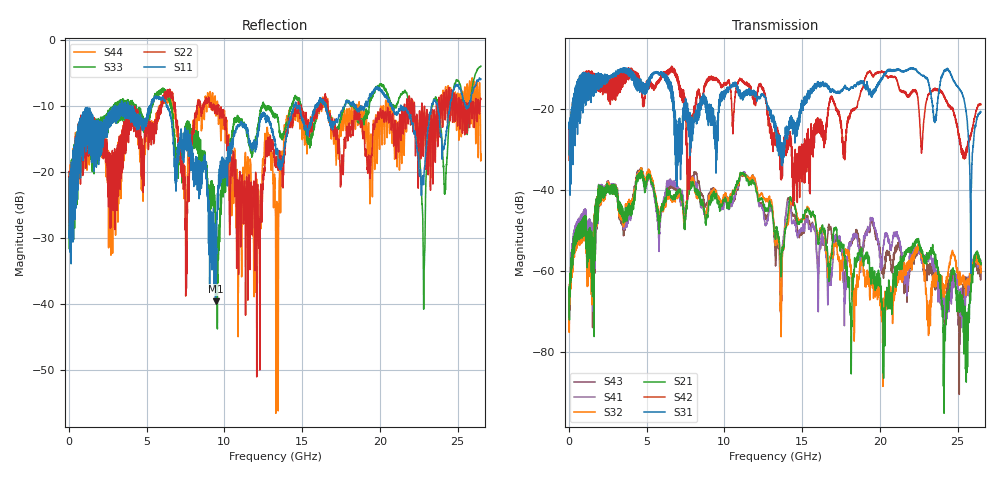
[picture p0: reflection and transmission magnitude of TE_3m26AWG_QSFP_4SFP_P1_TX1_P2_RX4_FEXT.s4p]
!Agilent Technologies,N5222A,MY51421691,A.10.00.00
!Agilent N5222A: A.10.00.00
!Date: Friday, January 30, 2015 12:38:07
!Correction: S11(Full 4 Port(1,2,3,4))
!S12(Full 4 Port(1,2,3,4))
!S13(Full 4 Port(1,2,3,4))
!S14(Full 4 Port(1,2,3,4))
!S21(Full 4 Port(1,2,3,4))
!S22(Full 4 Port(1,2,3,4))
!S23(Full 4 Port(1,2,3,4))
!S24(Full 4 Port(1,2,3,4))
!S31(Full 4 Port(1,2,3,4))
!S32(Full 4 Port(1,2,3,4))
!S33(Full 4 Port(1,2,3,4))
!S34(Full 4 Port(1,2,3,4))
!S41(Full 4 Port(1,2,3,4))
!S42(Full 4 Port(1,2,3,4))
!S43(Full 4 Port(1,2,3,4))
!S44(Full 4 Port(1,2,3,4))
!S4P File: Measurements: <S11,S12,S13,S14>,
!<S21,S22,S23,S24>,
!<S31,S32,S33,S34>,
!<S41,S42,S43,S44>:
# Hz S  dB  R 50.0
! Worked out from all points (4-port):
!   2650 points, 10 MHz to 26.5 GHz, reference 50 ohm
!   strongest paths, dB at 10 MHz, 6.63 GHz, 13.26 GHz, 19.88 GHz, 26.5 GHz:
!     S31: -24.8, -18.2, -24.4, -13.6, -20.8
!     S42: -25.1, -10.7, -25.1, -11.1, -19.0
!     S21: -64.0, -41.7, -51.8, -62.6, -58.5
!     S32: -65.0, -42.0, -53.0, -66.6, -58.4
!     S41: -67.7, -37.9, -51.4, -52.7, -57.5
!     S43: -70.9, -38.3, -56.2, -53.6, -59.5
!   lowest |S11| = -39.5 dB at 9.43 GHz (marker M1), VSWR 1.02, Z = 50.4 + j0.975 ohm
!   |S11| at or under -10 dB: start of sweep to 2.939 GHz; 6.343 GHz to 14.45 GHz (8.107 GHz wide, 78 % of centre); 21.36 GHz to 23.33 GHz (1.97 GHz wide, 8.82 % of centre)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
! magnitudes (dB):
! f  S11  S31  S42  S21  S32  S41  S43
! 10 MHz  -20.9  -24.8  -25.1  -64.0  -65.0  -67.7  -70.9
! 2.49 GHz  -11.6  -12.1  -13.2  -40.3  -39.3  -39.8  -39.1
! 7.7 GHz  -15.0  -22.6  -34.6  -40.9  -39.4  -40.1  -39.0
! 9.43 GHz  -39.5  -27.3  -12.3  -41.9  -41.3  -41.1  -40.7
! 14.52 GHz  -10.1  -23.6  -31.7  -44.1  -43.8  -48.4  -46.1
! 22.81 GHz  -21.9  -11.8  -23.6  -56.9  -59.3  -56.6  -59.5
! 26.5 GHz  -5.9  -20.8  -19.0  -58.5  -58.4  -57.5  -59.5
